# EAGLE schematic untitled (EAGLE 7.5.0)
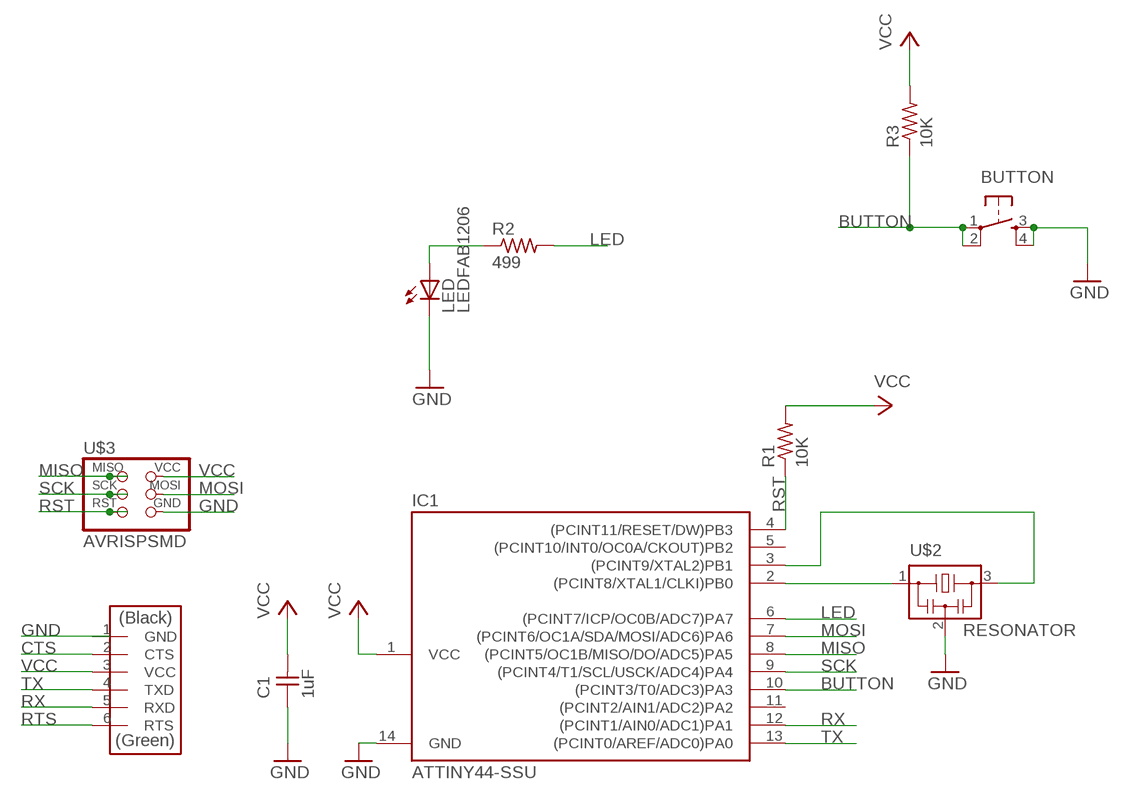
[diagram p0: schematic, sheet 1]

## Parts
BUTTON  6MM_SWITCH6MM_SWITCH  [6MM_SWITCH]
C1  1uF  CAP-UNPOLARIZEDFAB  [C1206FAB]
IC1  ATTINY44-SSU  [SOIC14]
LED  LEDFAB1206  [LED1206FAB]
R1  10K  RES-US1206FAB  [R1206FAB]
R2  499  RES-US1206FAB  [R1206FAB]
R3  10K  RES-US1206FAB  [R1206FAB]
U$2  RESONATOR  [EFOBM]
U$3  AVRISPSMD  [2X03SMD]
U$4  FTDI-SMD-HEADER  [1X06SMD]

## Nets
BUTTON: BUTTON.1(P) BUTTON.2(P1) IC1.10((PCINT3/T0/ADC3)PA3) R3.1
CTS: U$4.2(CTS)
GND: BUTTON.3(S) BUTTON.4(S1) C1.1 IC1.14(GND) LED.2(C) U$2.2 U$3.6(GND)
LED: IC1.6((PCINT7/ICP/OC0B/ADC7)PA7) R2.2
MISO: IC1.8((PCINT5/OC1B/MISO/DO/ADC5)PA5) U$3.1(MISO)
MOSI: IC1.7((PCINT6/OC1A/SDA/MOSI/ADC6)PA6) U$3.4(MOSI)
N$1: IC1.3((PCINT9/XTAL2)PB1) U$2.3
N$2: IC1.2((PCINT8/XTAL1/CLKI)PB0) U$2.1
N$3: LED.1(A) R2.1
RST: IC1.4((PCINT11/RESET/DW)PB3) R1.1 U$3.5(RST)
RTS: U$4.6(RTS)
RX: IC1.12((PCINT1/AIN0/ADC1)PA1) U$4.5(RXD)
SCK: IC1.9((PCINT4/T1/SCL/USCK/ADC4)PA4) U$3.3(SCK)
TX: IC1.13((PCINT0/AREF/ADC0)PA0) U$4.4(TXD)
VCC: C1.2 IC1.1(VCC) R1.2 R3.2 U$3.2(VCC) U$4.3(VCC)
Unconnected: IC1.5((PCINT10/INT0/OC0A/CKOUT)PB2) IC1.11((PCINT2/AIN1/ADC2)PA2) U$4.1(GND)

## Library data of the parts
BUTTON = fab:6MM_SWITCH: OMRON SWITCH
C1 = fab:CAP-UNPOLARIZED
IC1 = fab:ATTINY44
LED = fab:LED: LED
R1-R3 = fab:RES-US: Resistor (US Symbol)
U$2 = fab:RESONATOR
U$3 = fab:AVRISP
U$4 = fab:FTDI-SMD-HEADER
